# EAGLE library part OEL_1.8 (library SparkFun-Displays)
WiseChip SSD1320 - 1.80" Flexible Grayscale OLED 1.80" 160*32 pixel flexible grayscale OLED display
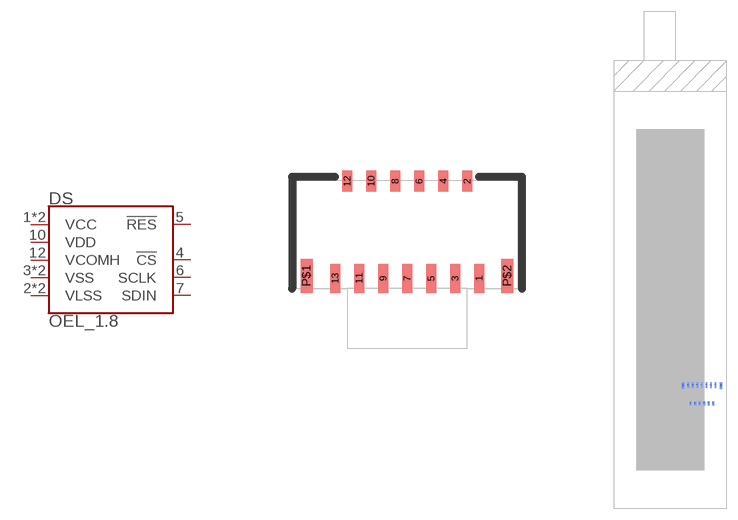
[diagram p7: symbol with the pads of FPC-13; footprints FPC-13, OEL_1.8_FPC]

Designator prefix DS

## OEL_1.8  [FPC-13]
1  VCC
2  VLSS
3  VSS
4  !CS!
5  !RES!
6  SCLK
7  SDIN
8  VSS
9  VLSS
10  VDD
12  VCOMH
13  VCC

## OEL_1.8OEL_1.8  [OEL_1.8_FPC]
Pads as for FPC-13

## OEL_1.8-AYF331335  [AYF331335]
1  VCC
2  VCOMH
4  VDD
5  VLSS
6  VSS
7  SDIN
8  SCLK
9  !RES!
10  !CS!
11  VSS
12  VLSS
13  VCC

## OEL_1.8OEL_Y3B (PROD_ID: LCD-13910, CONN-13933)  [OEL_1.8_FPC_Y3B]
Pads as for FPC-13

## Footprint FPC-13 (pad centres in mm)
FPC Connector - 13 Pin Example Datasheet
smd 0.25 x 0.72: 1 1.8,-1.265; 3 1.2,-1.265; 5 0.6,-1.265; 7 0,-1.265; 9 -0.6,-1.265; 11 -1.2,-1.265; 13 -1.8,-1.265
smd 0.25 x 0.52: 2 1.5,1.165; 4 0.9,1.165; 6 0.3,1.165; 8 -0.3,1.165; 10 -0.9,1.165; 12 -1.5,1.165
smd 0.3 x 0.85: P$1 -2.51,-1.2; P$2 2.51,-1.2

## Footprint OEL_1.8_FPC (pad centres in mm)
1.81" Greyscale OLED Includes FPC connector on bottom side and dimensions of display. bDoc outline indicates approximate location of the FPC cable.
smd 0.25 x 0.72 bottom: 1 6,-11.32; 3 5.4,-11.32; 5 4.8,-11.32; 7 4.2,-11.32; 9 3.6,-11.32; 11 3,-11.32; 13 2.4,-11.32
smd 0.25 x 0.52 bottom: 2 5.7,-13.75; 4 5.1,-13.75; 6 4.5,-13.75; 8 3.9,-13.75; 10 3.3,-13.75; 12 2.7,-13.75
smd 0.3 x 0.85 bottom: P$1 1.69,-11.385; P$2 6.71,-11.385

## Footprint AYF331335 (pad centres in mm)
Panasonic Y3B FPC Connector - 13 Pin Low-profile, top/bottom contact connector for 13-pin, 0.3mm pitch FPC connector. Datasheet
smd 0.23 x 0.44: 1 -1.8,1.355; 3 -1.2,1.355; 5 -0.6,1.355; 7 0,1.355; 9 0.6,1.355; 11 1.2,1.355; 13 1.8,1.355
smd 0.23 x 0.34: 2 -1.5,-1.405; 4 -0.9,-1.405; 6 -0.3,-1.405; 8 0.3,-1.405; 10 0.9,-1.405; 12 1.5,-1.405

## Footprint OEL_1.8_FPC_Y3B (pad centres in mm)
1.81" Greyscale OLED Includes Panasonic Y3B FPC connector on bottom side and dimensions of display. bDoc outline indicates approximate location of the FPC cable. Specifications: Pin count: 13 Pin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
smd 0.23 x 1 bottom: 1 6,-11.795; 2 5.7,-14.955; 3 5.4,-11.795; 4 5.1,-14.955; 5 4.8,-11.795; 6 4.5,-14.955; 7 4.2,-11.795; 8 3.9,-14.955; 9 3.6,-11.795; 10 3.3,-14.955; 11 3,-11.795; 12 2.7,-14.955; 13 2.4,-11.795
